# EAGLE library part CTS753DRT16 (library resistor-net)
Network Resistor CTS 753 Series Leadless Surface Mount Source: http://www.ctscorp.com/components/Datasheets/753.pdf Distributor: Digi Key
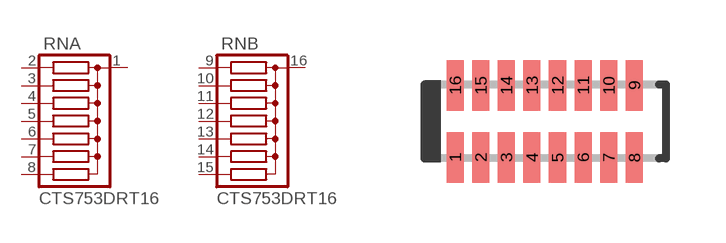
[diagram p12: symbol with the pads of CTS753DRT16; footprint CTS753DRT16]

Designator prefix RN; gates A=RN1X7 B=RN1X7

## CTS753DRT16 (OC_FARNELL: unknown; OC_NEWARK: unknown)  [CTS753DRT16]
1  A:C  pas
2  A:1  pas
3  A:2  pas
4  A:3  pas
5  A:4  pas
6  A:5  pas
7  A:6  pas
8  A:7  pas
9  B:1  pas
10  B:2  pas
11  B:3  pas
12  B:4  pas
13  B:5  pas
14  B:6  pas
15  B:7  pas
16  B:C  pas

## Footprint CTS753DRT16 (pad centres in mm)
Network Resistor Leadless Surface Mount Series 753 Source: http://www.ctscorp.com/components/Datasheets/753.pdf
smd 0.43 x 1.27: 1 -2.24,-0.9; 2 -1.6,-0.9; 3 -0.96,-0.9; 4 -0.32,-0.9; 5 0.32,-0.9; 6 0.96,-0.9; 7 1.6,-0.9; 8 2.24,-0.9; 9 2.24,0.9; 10 1.6,0.9; 11 0.96,0.9; 12 0.32,0.9; 13 -0.32,0.9; 14 -0.96,0.9; 15 -1.6,0.9; 16 -2.24,0.9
